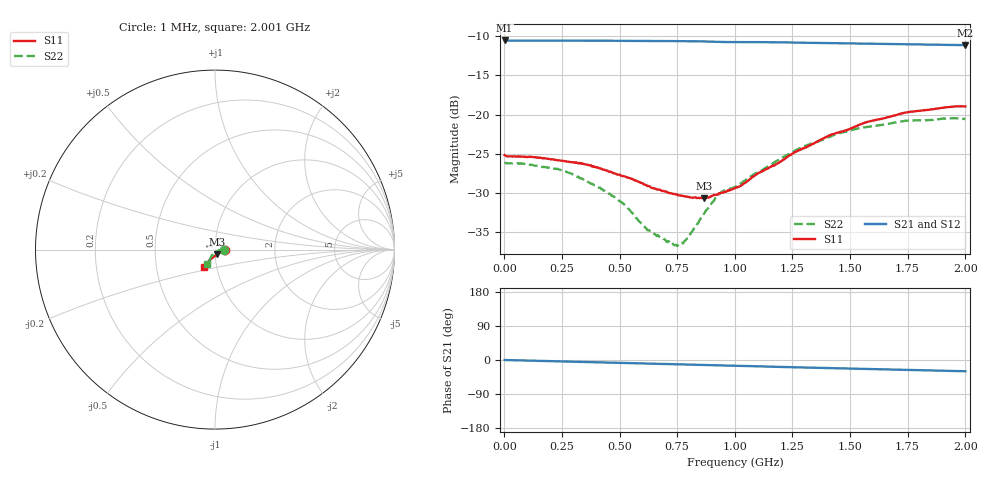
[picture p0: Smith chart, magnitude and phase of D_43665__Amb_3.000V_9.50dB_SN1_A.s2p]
! device id: 43665_
! dir: \\malibu\benchdata\1_engineers\tn_data\43665_75ohm\new\sparar\43665_\amb\3p000v\9p50db
! Serial: 1
! Insertion: A
! Temp: Amb
! VDD: 3.000V
! Attenuation Step: 9.50dB
! IDD: 1.453747e+00mA
! FILE NAME
! DATE 03-27-2009 08:35:41
! CORRECTED  DATA
#  Hz  S  RI  R  75
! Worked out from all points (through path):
!   401 points, 1 MHz to 2.001 GHz, reference 75 ohm
!   highest |S21| = -10.52 dB at 1 MHz (marker M1); lowest = -11.1 dB at 2.001 GHz (marker M2)
!   group delay of S21, straight-line fit = 42 ps
!   lowest |S11| = -30.7 dB at 866 MHz (marker M3), VSWR 1.06, Z = 77 - j3.96 ohm
!   |S11| at or under -10 dB: start of sweep to end of sweep
!   |S22| runs from -36.9 to -20.5 dB; largest |S21 - S12| = 0.0012
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1000000  0.055 -0.000485  0.2979 -0.00042  0.298 -0.000582  0.0493 -0.000547
2.31e8  0.0507 -0.00295  0.2967 -0.0175  0.2968 -0.0176  0.0448 0.00289
3.36e8  0.0485 -0.00535  0.2959 -0.0257  0.2959 -0.0257  0.0387 0.00326
4.26e8  0.0439 -0.00698  0.295 -0.0326  0.295 -0.0327  0.0331 0.00133
5.11e8  0.0392 -0.00979  0.2938 -0.0394  0.2938 -0.0394  0.0272 -0.00117
6.11e8  0.0329 -0.0134  0.2918 -0.047  0.2919 -0.047  0.0184 -0.00437
6.71e8  0.0288 -0.0162  0.2909 -0.0517  0.2909 -0.0517  0.0146 -0.00792
7.41e8  0.0241 -0.0194  0.2894 -0.0573  0.2895 -0.0573  0.00918 -0.0113
7.71e8  0.0218 -0.0208  0.2886 -0.0597  0.2887 -0.0597  0.00644 -0.0136
7.96e8  0.02 -0.022  0.288 -0.0618  0.288 -0.0617  0.00421 -0.0155
8.66e8  0.0136 -0.0257  0.2858 -0.0676  0.2857 -0.0675  -0.00144 -0.0231
9.36e8  0.00712 -0.0305  0.2824 -0.0725  0.2825 -0.0723  -0.01 -0.0295
1.001e9  0.00209 -0.0337  0.281 -0.0758  0.2812 -0.0757  -0.017 -0.0298
1.211e9  -0.0176 -0.0483  0.2748 -0.0917  0.2752 -0.0916  -0.0247 -0.0475
1.261e9  -0.0225 -0.0527  0.2726 -0.0952  0.273 -0.0952  -0.0272 -0.0519
1.336e9  -0.0282 -0.0581  0.2698 -0.1  0.2703 -0.1  -0.0307 -0.0578
1.411e9  -0.0349 -0.0648  0.2668 -0.1054  0.2673 -0.1056  -0.0316 -0.0645
1.511e9  -0.0422 -0.0706  0.2624 -0.1114  0.2629 -0.1116  -0.0372 -0.0707
1.576e9  -0.0469 -0.0765  0.2597 -0.1153  0.2603 -0.1159  -0.038 -0.0742
1.671e9  -0.0519 -0.0814  0.2556 -0.1208  0.2557 -0.1213  -0.0407 -0.0773
1.756e9  -0.0559 -0.0876  0.252 -0.1255  0.2522 -0.1263  -0.0418 -0.0815
2.001e9  -0.061 -0.0947  0.2415 -0.1377  0.2406 -0.1385  -0.0457 -0.0814
